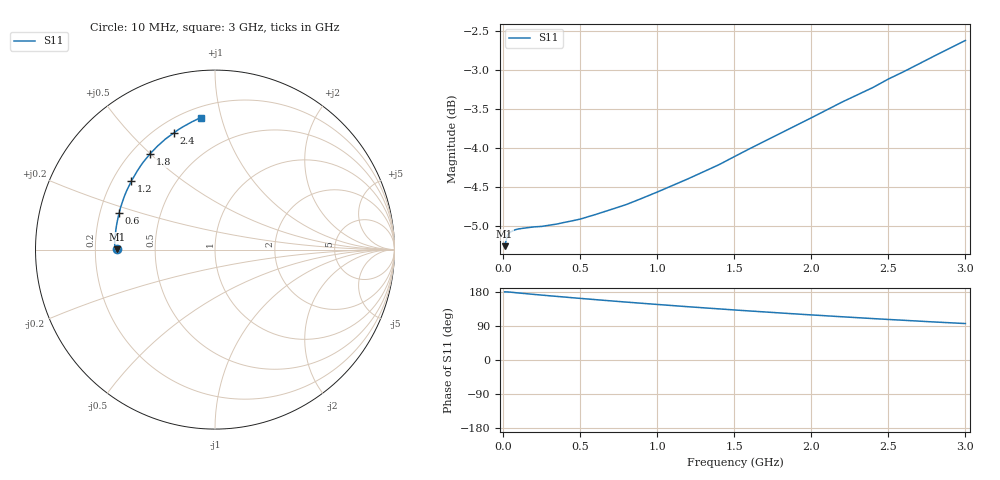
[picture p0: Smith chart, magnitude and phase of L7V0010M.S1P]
! SIEMENS Small Signal Semiconductors
! BAR14-1
! Si PIN Diode in SOT23
! IF = 10 mA
! S-Parameters:  July  1992
# GHz  S  MA  R  50
!  f  S11
! GHz  MAG  ANG
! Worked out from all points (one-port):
!   31 points, 10 MHz to 3 GHz, reference 50 ohm
!   lowest |S11| = -5.3 dB at 10 MHz (marker M1), VSWR 3.40, Z = 14.7 + j0.0399 ohm
!   |S11| at or under -10 dB: nowhere
!   S11 on the Smith chart (normalised r, x): 10 MHz: 0.29, +0.00; 600 MHz: 0.28, +0.17; 1.2 GHz: 0.28, +0.33; 1.8 GHz: 0.27, +0.50; 2.4 GHz: 0.27, +0.67; 3 GHz: 0.27, +0.86
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0.01  0.5455 179.9
0.03  0.5549 179.6
0.05  0.5572 179.0
0.06  0.5579 178.5
0.08  0.559 177.7
0.1  0.5596 176.9
0.15  0.5605 175.0
0.2  0.5613 173.1
0.3  0.5627 169.5
0.4  0.5651 166.1
0.45  0.5664 164.3
0.6  0.5717 159.3
0.7  0.5759 156.0
0.8  0.5802 152.8
0.9  0.5855 149.7
1  0.591 146.6
1.2  0.6027 140.6
1.4  0.6154 134.9
1.5  0.6228 132.1
1.6  0.6302 129.4
1.8  0.6448 124.1
2  0.6597 119.0
2.2  0.6753 114.1
2.4  0.69 109.3
2.5  0.6987 107.0
2.6  0.7064 104.8
2.8  0.7231 100.3
3  0.7398 96.2
